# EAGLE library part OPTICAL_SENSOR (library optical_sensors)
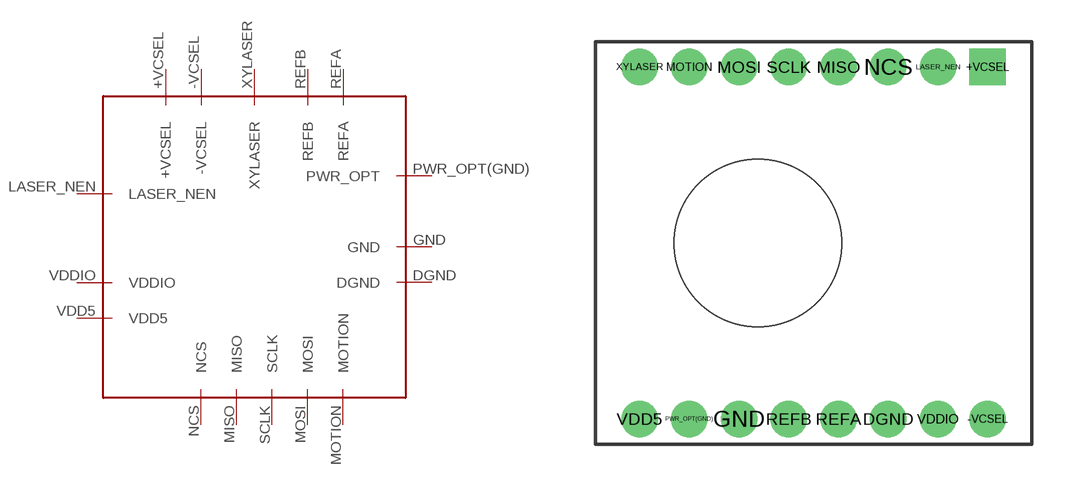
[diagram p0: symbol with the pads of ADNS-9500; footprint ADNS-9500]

Designator prefix -

## OPTICAL_SENSOR  [ADNS-9500]
+VCSEL  +VCSEL
-VCSEL  -VCSEL
DGND  DGND
GND  GND
LASER_NEN  LASER_NEN
MISO  MISO
MOSI  MOSI
MOTION  MOTION
NCS  NCS
PWR_OPT(GND)  PWR_OPT
REFA  REFA
REFB  REFB
SCLK  SCLK
VDD5  VDD5
VDDIO  VDDIO
XYLASER  XYLASER

## Footprint ADNS-9500 (pad centres in mm)
drill 0.8 square: +VCSEL 6.23,6.3
drill 0.8: -VCSEL 6.23,-6.3; DGND 2.67,-6.3; GND -2.67,-6.3; LASER_NEN 4.45,6.3; MISO 0.89,6.3; MOSI -2.67,6.3; MOTION -4.45,6.3; NCS 2.67,6.3; PWR_OPT(GND) -4.45,-6.3; REFA 0.89,-6.3; REFB -0.89,-6.3; SCLK -0.89,6.3; VDD5 -6.23,-6.3; VDDIO 4.45,-6.3; XYLASER -6.23,6.3
hole 6 at -2,0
